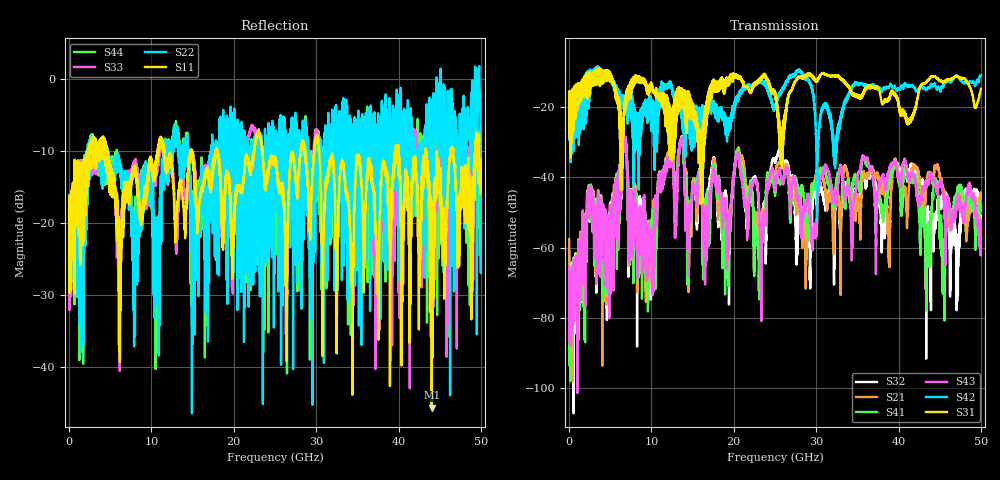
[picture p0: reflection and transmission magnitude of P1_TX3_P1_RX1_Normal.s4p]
!Keysight Technologies,N5225B,MY57041031,A.13.20.10
!Date: Friday, May 31, 2019 11:13:55
!Correction: S11(Full 4 Port(1,2,3,4))
!S12(Full 4 Port(1,2,3,4))
!S13(Full 4 Port(1,2,3,4))
!S14(Full 4 Port(1,2,3,4))
!S21(Full 4 Port(1,2,3,4))
!S22(Full 4 Port(1,2,3,4))
!S23(Full 4 Port(1,2,3,4))
!S24(Full 4 Port(1,2,3,4))
!S31(Full 4 Port(1,2,3,4))
!S32(Full 4 Port(1,2,3,4))
!S33(Full 4 Port(1,2,3,4))
!S34(Full 4 Port(1,2,3,4))
!S41(Full 4 Port(1,2,3,4))
!S42(Full 4 Port(1,2,3,4))
!S43(Full 4 Port(1,2,3,4))
!S44(Full 4 Port(1,2,3,4))
!S4P File: Measurements: <S11,S12,S13,S14>,
!<S21,S22,S23,S24>,
!<S31,S32,S33,S34>,
!<S41,S42,S43,S44>:
# Hz S  dB  R 50.0
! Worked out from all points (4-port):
!   5000 points, 10 MHz to 50 GHz, reference 50 ohm
!   strongest paths, dB at 10 MHz, 12.51 GHz, 25.01 GHz, 37.51 GHz, 50 GHz:
!     S31: -19.3, -27.2, -15.7, -14.5, -14.9
!     S42: -19.5, -14.8, -19.9, -15.2, -11.1
!     S43: -65.5, -34.6, -43.2, -43.8, -56.5
!     S41: -71.6, -33.4, -45.4, -45.4, -49.6
!     S21: -57.6, -31.6, -39.6, -39.6, -45.0
!     S32: -61.0, -32.8, -35.8, -44.7, -54.5
!   lowest |S11| = -45.6 dB at 44.03 GHz (marker M1), VSWR 1.01, Z = 49.9 + j0.51 ohm
!   |S11| at or under -10 dB: 4.66 GHz to 10.77 GHz (6.106 GHz wide, 79.2 % of centre); 23.49 GHz to 28.08 GHz (4.585 GHz wide, 17.8 % of centre); 30.37 GHz to 39.61 GHz (9.241 GHz wide, 26.4 % of centre)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
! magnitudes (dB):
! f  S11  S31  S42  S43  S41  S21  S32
! 10 MHz  -19.5  -19.3  -19.5  -65.5  -71.6  -57.6  -61.0
! 6.75 GHz  -15.8  -20.1  -21.1  -29.8  -29.7  -30.2  -30.2
! 9.89 GHz  -10.8  -14.9  -17.1  -57.4  -54.1  -62.5  -68.1
! 13.66 GHz  -15.0  -19.8  -20.6  -28.9  -29.4  -29.3  -28.8
! 23.37 GHz  -8.9  -11.5  -13.4  -63.8  -55.9  -51.6  -60.0
! 44.03 GHz  -45.6  -11.4  -13.7  -39.5  -49.2  -39.9  -54.1
! 50 GHz  -12.3  -14.9  -11.1  -56.5  -49.6  -45.0  -54.5
